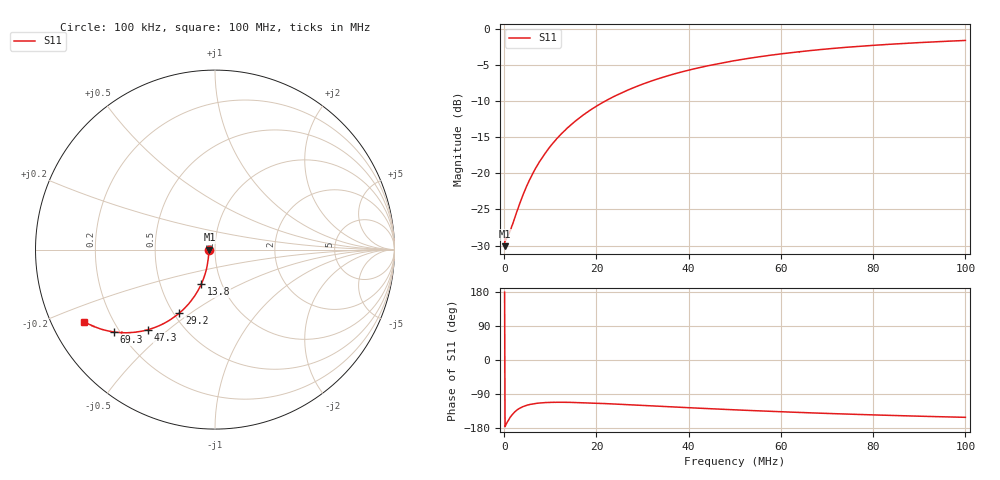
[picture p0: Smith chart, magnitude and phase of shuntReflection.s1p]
# Hz S RI R 50.0
! written by SimSmith version 18.3h
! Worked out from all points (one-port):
!   1000 points, 100 kHz to 100 MHz, reference 50 ohm
!   lowest |S11| = -30.1 dB at 100 kHz (marker M1), VSWR 1.06, Z = 47 + j0.0463 ohm
!   |S11| at or under -10 dB: start of sweep to 21.87 MHz
!   S11 on the Smith chart (normalised r, x): 100 kHz: 0.94, +0.00; 13.8 MHz: 0.80, -0.32; 29.2 MHz: 0.53, -0.45; 47.3 MHz: 0.32, -0.43; 69.3 MHz: 0.18, -0.35; 100 MHz: 0.10, -0.25
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100000  -0.0313 0.000493
700000  -0.0349 -0.00998
1400000  -0.0351 -0.0203
3100000  -0.037 -0.045
4400000  -0.0394 -0.0641
5300000  -0.0412 -0.0768
6200000  -0.0435 -0.0897
7600000  -0.0479 -0.1096
9000000  -0.0531 -0.1289
1.07e7  -0.0608 -0.1521
1.26e7  -0.07 -0.1773
1.38e7  -0.0769 -0.193
1.63e7  -0.0924 -0.2241
1.89e7  -0.111 -0.2543
2.18e7  -0.1335 -0.2857
2.51e7  -0.1616 -0.3184
2.92e7  -0.1988 -0.3538
3.31e7  -0.2365 -0.3824
3.76e7  -0.2805 -0.409
4.22e7  -0.3258 -0.43
4.73e7  -0.3749 -0.4465
5.01e7  -0.4012 -0.4531
5.58e7  -0.4525 -0.4608
6.26e7  -0.5095 -0.4628
6.93e7  -0.5611 -0.4592
7.51e7  -0.6002 -0.4522
8.76e7  -0.6735 -0.4292
1e8  -0.7315 -0.4008
